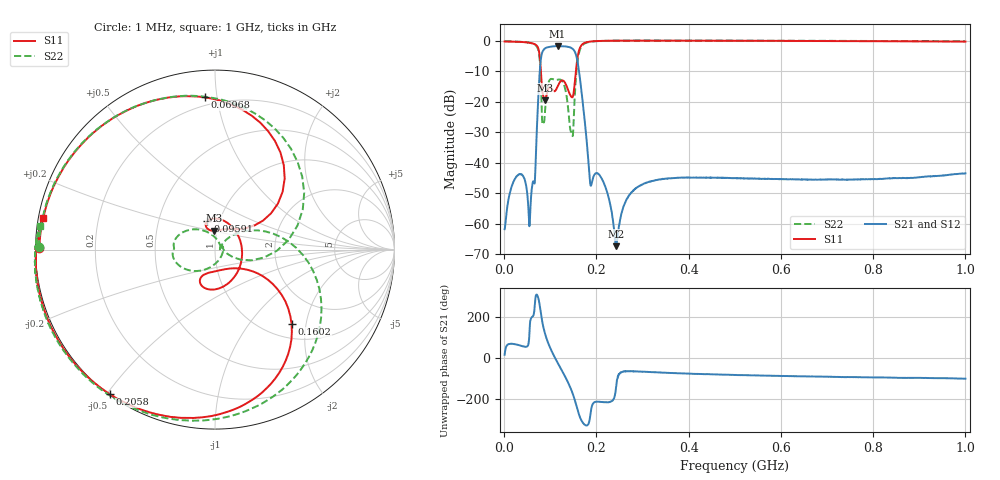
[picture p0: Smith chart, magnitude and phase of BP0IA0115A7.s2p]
!Agilent Technologies,E8358A,US41080443,A.07.50.56
!Agilent E8358A: A.07.50.56
!Date: Tuesday, October 31, 2017 22:05:40
!Correction: S11(Full 2 Port(1,2))
!S21(Full 2 Port(1,2))
!S12(Full 2 Port(1,2))
!S22(Full 2 Port(1,2))
!S2P File: Measurements: S11, S21, S12, S22:
# Hz S  dB  R 50
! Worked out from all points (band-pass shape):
!   1601 points, 1 MHz to 1 GHz, reference 50 ohm
!   highest |S21| = -1.70 dB at 115.9 MHz (marker M1); lowest = -67.4 dB at 243.3 MHz (marker M2)
!   |S21| within 3 dB of the highest: 80.97 MHz to 156 MHz (75 MHz wide, 63.3 % of centre)
!   lowest |S11| = -19.6 dB at 88.41 MHz (marker M3), VSWR 1.23, Z = 48.4 + j10.3 ohm
!   |S11| at or under -10 dB: 79.63 MHz to 155.4 MHz (75.8 MHz wide, 64.5 % of centre)
!   |S22| runs from -31.3 to 0.1 dB; largest |S21 - S12| = 0.0036
!   S11 on the Smith chart (normalised r, x): 1 MHz: 0.01, +0.01; 69.68 MHz: 0.15, +0.92; 95.91 MHz: 0.88, +0.28; 160.2 MHz: 1.30, -1.65; 205.8 MHz: 0.00, -0.51; 1 GHz: 0.01, +0.09
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1000000  -0.19 179.4  -61.85 15.3  -62.17 15.1  -0.16 179.3
3.034562e7  -0.30 158.7  -44.01 62.9  -43.92 63.0  -0.28 158.3
5.5945e7  -0.63 129.4  -58.49 164.8  -58.27 165.8  -0.66 127.1
6.968125e7  -1.41 93.8  -33.71 -54.4  -33.71 -54.0  -1.66 84.2
7.84225e7  -7.26 36.1  -7.62 -125.2  -7.59 -125.0  -9.24 -1.0
8.404188e7  -17.54 60.1  -3.30 158.8  -3.28 158.9  -26.73 23.6
8.84125e7  -19.59 92.7  -2.50 119.1  -2.47 119.3  -23.60 -75.5
9.5905e7  -15.71 105.0  -2.05 69.4  -2.01 69.5  -13.83 -149.1
1.15885e8  -14.95 -47.0  -1.70 -23.2  -1.70 -23.3  -12.77 176.3
1.321188e8  -13.78 -113.8  -1.82 -89.6  -1.83 -89.5  -15.63 137.0
1.45855e8  -18.39 -88.0  -2.33 -156.0  -2.34 -155.9  -30.06 -7.9
1.602156e8  -4.52 -44.1  -7.83 100.8  -7.87 101.1  -5.57 -8.0
1.677081e8  -1.41 -73.7  -16.61 57.2  -16.63 57.5  -1.83 -51.9
1.870638e8  -0.23 -110.2  -47.28 86.5  -47.35 87.1  -0.28 -100.8
2.05795e8  -0.03 -126.0  -43.93 148.2  -43.86 148.3  -0.03 -120.5
2.432575e8  0.06 -142.5  -67.44 -134.7  -66.99 -136.6  0.10 -139.5
2.719788e8  0.08 -149.8  -50.52 -63.8  -50.47 -63.6  0.12 -147.6
3.344162e8  0.08 -159.8  -45.56 -70.2  -45.60 -70.1  0.12 -158.1
5.005e8  0.03 -172.8  -45.06 -82.4  -45.08 -82.2  0.08 -171.4
6.672081e8  -0.03 179.9  -45.57 -89.7  -45.61 -89.7  0.02 -178.6
8.339162e8  -0.13 174.3  -45.15 -94.3  -45.17 -95.0  -0.05 176.4
1e9  -0.24 169.5  -43.51 -100.2  -43.50 -100.1  -0.14 172.3
